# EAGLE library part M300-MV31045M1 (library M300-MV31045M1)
Headers & Wire Housings 10 WAY MALE PC TAIL DIL WJS Source: Datasheet
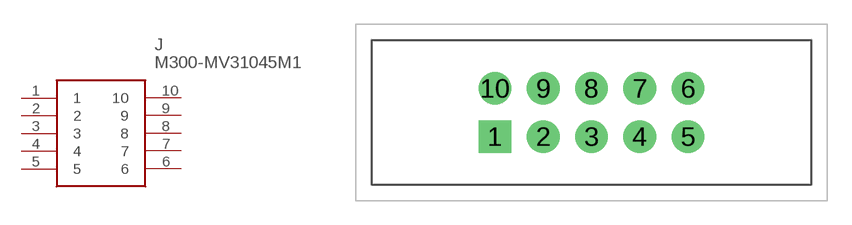
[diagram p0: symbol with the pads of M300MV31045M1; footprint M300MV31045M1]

Designator prefix J

## M300-MV31045M1 (Description: Headers & Wire Housings 10 WAY MALE PC TAIL DIL WJS; Height: 7.05mm; Manufacturer_Name: HARWIN; Manufacturer_Part_Number: M300-MV31045M1)  [M300MV31045M1]
1  1
2  2
3  3
4  4
5  5
6  6
7  7
8  8
9  9
10  10

## Footprint M300MV31045M1 (pad centres in mm)
M300-MV31045M1-1
drill 1.35 pad 2.025 square: 1 0,0
drill 1.35 pad 2.025: 2 3,0; 3 6,0; 4 9,0; 5 12,0; 6 12,3; 7 9,3; 8 6,3; 9 3,3; 10 0,3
